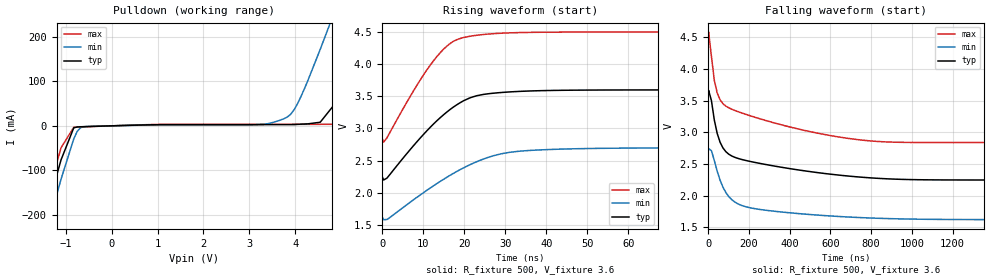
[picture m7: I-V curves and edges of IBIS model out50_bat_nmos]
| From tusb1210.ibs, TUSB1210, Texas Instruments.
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|   Model: out50_bat_nmos
|   Description:  Output buffer under VBAT NMOS enabled
[Model]   out50_bat_nmos
Model_type   Open_drain
Polarity   Non-Inverting
Vmeas =   1.800
Vref =   3.6
Cref =   5e-12
Rref =   2.7e3
|variable   typ   min   max
C_comp   0.087p   0.067p   0.184p
[Temperature Range]   27   125   -40
[Voltage Range]   3.6   2.7   4.5
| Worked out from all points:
|   slope of the pulldown table from 0 to 0.54 V, typ, clamps not added: 348 ohm
|   rising waveform, R_fixture 500, V_fixture 3.6: 20-80 % time 12.5ns typ, 16.7ns min, 10.1ns max; typ from 2.25 V to 3.6 V
|   falling waveform, R_fixture 500, V_fixture 3.6: 20-80 % time 217ns typ, 137ns min, 283ns max; typ from 3.6 V to 2.25 V
[Pulldown]
| out50_bat_nmos
|Voltage   I(typ)   I(min)   I(max)
-3.6V     -1.024A    -1.054A    -1.007A
-1.657V   -284.2mA   -326.5mA   -257.6mA
-1.38V    -178.7mA   -222.5mA   -151.2mA
-825mV    -4.513mA   -29.35mA   -3.185mA
3.675V    2.714mA    12.97mA    3.328mA
3.975V    2.963mA    36.45mA    3.331mA
4.541V    8.028mA    171.5mA    3.34mA
4.807V    42.23mA    243.7mA    3.391mA
5.339V    181.9mA    391.8mA    6.359mA
5.604V    256.7mA    467mA      34.86mA
6.402V    488.4mA    724.8mA    255.5mA
7.2V      776.3mA    1.027A     498.3mA
[Ramp]
| out50_bat_nmos
|variable   typ   min   max
dV/dt_r   0.495/2.724e-08   0.292/3.991e-08   0.726/2.128e-08
dV/dt_f   1.355/7.311e-07   1.082/7.070e-07   1.662/6.895e-07
R_load =   50
[Rising Waveform]
| out50_bat_nmos
R_fixture =   500
V_fixture =   3.6
V_fixture_min =   2.7
V_fixture_max =   4.5
|Time   V(typ)   V(min)   V(max)
0s        2.245V     1.618V     2.838V
310.7ps   2.198V     1.582V     2.786V
1.123ns   2.228V     1.585V     2.853V
8.438ns   2.792V     1.929V     3.67V
13.31ns   3.119V     2.143V     4.116V
17.38ns   3.333V     2.303V     4.354V
21.44ns   3.476V     2.437V     4.431V
30.38ns   3.563V     2.621V     4.482V
43.39ns   3.591V     2.678V     4.495V
161.3ns   3.598V     2.698V     4.498V
[Falling Waveform]
| out50_bat_nmos
R_fixture =   500
V_fixture =   3.6
V_fixture_min =   2.7
V_fixture_max =   4.5
|Time   V(typ)   V(min)   V(max)
0s        3.6V       2.7V       4.5V
1.974ns   3.663V     2.742V     4.586V
16.03ns   3.499V     2.708V     4.197V
30.08ns   3.193V     2.553V     3.821V
44.13ns   2.982V     2.386V     3.623V
86.29ns   2.695V     2.05V      3.414V
198.7ns   2.544V     1.812V     3.269V
578.1ns   2.346V     1.682V     2.961V
957.6ns   2.255V     1.63V      2.841V
2.786us   2.245V     1.618V     2.838V
